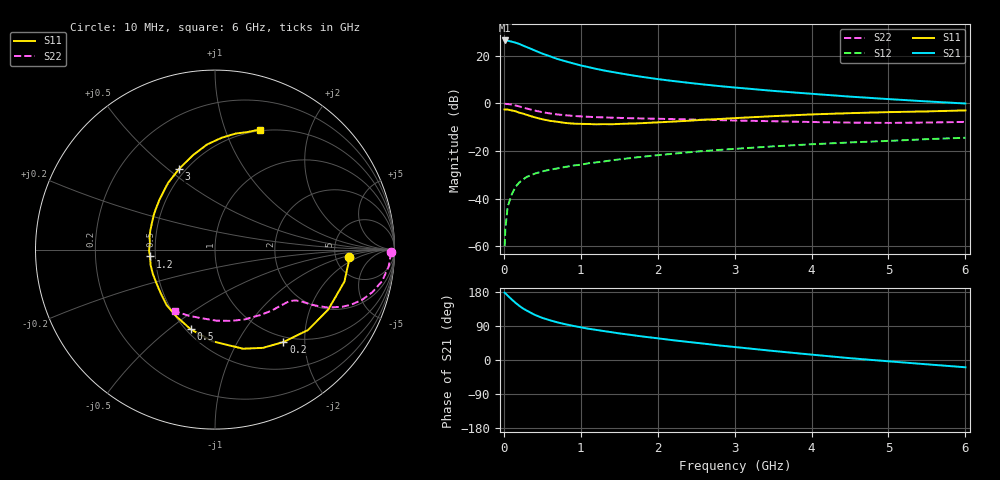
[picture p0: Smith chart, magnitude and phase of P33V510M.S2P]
! SIEMENS Small Signal Semiconductors
! BFP181
! Si NPN RF Bipolar Junction Transistor in SOT143
! VCE = 3.5 V  IC = 10 mA
! Common Emitter S-Parameters:  March  1996
# GHz  S  MA  R  50
!  f  S11  S21  S12  S22
! GHz  MAG  ANG  MAG  ANG  MAG  ANG  MAG  ANG
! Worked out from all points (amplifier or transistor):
!   36 points, 10 MHz to 6 GHz, reference 50 ohm
!   highest |S21| = 26.5 dB at 10 MHz (marker M1)
!   |S21| within 3 dB of that: start of sweep to 313.2 MHz
!   unconditionally stable (mu >= 1): 1.162 GHz to 5.998 GHz
!   at 250 MHz: K = 0.34, MSG = 28.1 dB, |S12| = -31.9 dB
!   at 1.4 GHz: K = 1.07, MAG = 16.9 dB, |S12| = -23.9 dB
!   at 6 GHz: K = 1.00, MSG = 7.2 dB, |S12| = -14.4 dB
!   S11 on the Smith chart (normalised r, x): 10 MHz: 6.61, -1.24; 200 MHz: 0.91, -1.59; 500 MHz: 0.53, -0.60; 1.2 GHz: 0.47, -0.04; 3 GHz: 0.46, +0.55; 6 GHz: 0.49, +1.32
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0.01  0.7452 -3.2  21.07 177.7  0.001 74.2  0.9803 -0.9
0.02  0.7473 -5.8  20.94 176.2  0.0023 88.4  0.9786 -2.1
0.05  0.7428 -13.9  20.82 169.8  0.0068 86.4  0.9723 -5.5
0.1  0.7139 -27.9  19.95 160.3  0.0119 76.0  0.9475 -10.7
0.15  0.6849 -40.9  18.96 151.2  0.0175 69.5  0.9087 -15.1
0.2  0.6407 -53.5  17.83 143.0  0.0218 65.4  0.8656 -18.9
0.25  0.6091 -64.0  16.43 135.8  0.0253 61.7  0.82 -21.9
0.3  0.5739 -74.2  15.22 130.2  0.0287 58.5  0.7795 -24.1
0.4  0.5111 -91.6  13.02 119.3  0.0334 54.5  0.7091 -27.1
0.5  0.4639 -107.0  11.15 111.1  0.0373 51.5  0.6546 -28.7
0.6  0.4309 -119.6  9.786 104.8  0.0405 50.2  0.6156 -29.8
0.7  0.4108 -131.0  8.554 99.2  0.0432 49.4  0.586 -30.4
0.9  0.3765 -149.8  6.95 90.2  0.0494 48.6  0.5481 -31.5
1.1  0.3691 -166.6  5.799 82.5  0.0552 49.0  0.5237 -32.8
1.2  0.3637 -174.0  5.331 79.5  0.0577 48.5  0.5157 -33.6
1.7  0.3796 158.8  3.82 64.8  0.0728 48.3  0.4879 -38.6
2.2  0.4155 138.3  2.96 52.2  0.0875 46.2  0.4685 -45.1
3  0.4913 114.2  2.163 34.3  0.1111 41.5  0.4374 -57.7
3.5  0.5403 103.1  1.837 23.9  0.1251 38.2  0.4224 -67.1
4.5  0.6247 86.5  1.39 4.8  0.1513 30.5  0.3959 -88.7
5.5  0.6798 74.5  1.103 -11.4  0.1774 23.4  0.3965 -111.6
6  0.7135 69.6  0.997 -19.2  0.1902 19.4  0.4095 -123.2
